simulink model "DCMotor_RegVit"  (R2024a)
settings: Solver=ode45  StartTime=0.0  StopTime=6  FixedStep=TE/100  RelTol=1e-3
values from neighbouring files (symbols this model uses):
  Ki = 0    [Constants_RegVit.m]
  Kp = 0    [Constants_RegVit.m]
  Kwc1 = 0    [Constants_RegVit.m]
  Kwc2 = 0    [Constants_RegVit.m]
  LIMREG = 0    [Constants_RegVit.m]
  TE = 0    [Constants_RegVit.m]
  TM = 0    [Constants_RegVit.m]
  TpE = 0    [Constants_RegVit.m]

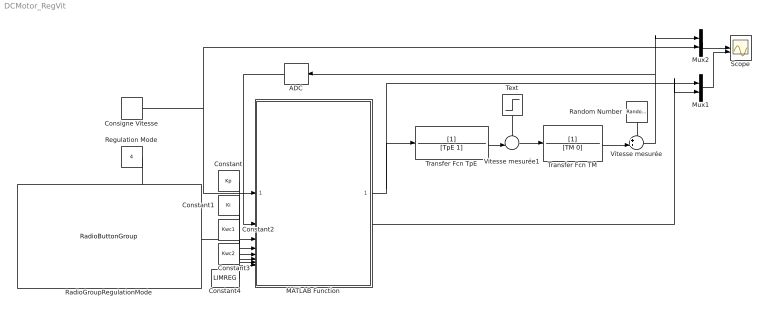
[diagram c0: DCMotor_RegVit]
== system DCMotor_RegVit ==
  ADC : ZeroOrderHold  SampleTime=TE
  Consigne Vitesse : DiscretePulseGenerator  Period=3/TE  PulseWidth=3/(2*TE)  SampleTime=TE
  Constant : Constant  Value=Kp
  Constant1 : Constant  Value=Ki
  Constant2 : Constant  Value=Kwc1
  Constant3 : Constant  Value=Kwc2
  Constant4 : Constant  Value=LIMREG
  MATLAB Function : MATLAB Function  TreatAsAtomicUnit=on
  Mux1 : Mux  Inputs=2
  Mux2 : Mux  Inputs=2
  RadioGroupRegulationMode : RadioButtonGroup  LabelPosition=Hide  SelectedLabel=THEORETICAL  ButtonGroupName=Regulation Mode
  Random Number : RandomNumber  Variance=0.00005  SampleTime=TE
  Regulation Mode : Constant  Value=4
  Scope : Scope  NumInputPorts=2
  Text : Step  Time=4  SampleTime=0
  Transfer Fcn TM : TransferFcn  Denominator=[TM 0]
  Transfer Fcn TpE : TransferFcn  Denominator=[TpE 1]
  Vitesse mesurée : Sum  Inputs=++|
  Vitesse mesurée1 : Sum  Inputs=-+|
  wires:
  Mux2/1 -> Scope/1
  Consigne Vitesse/1 -> Mux2/2, MATLAB Function/1(speedSetValue)
  Transfer Fcn TM/1 -> Vitesse mesurée/2
  Vitesse mesurée/1 -> Mux2/1, ADC/1
  Random Number/1 -> Vitesse mesurée/1
  ADC/1 -> MATLAB Function/2(speedMeasure)
  MATLAB Function/1(regOutLim) -> Mux1/1, Transfer Fcn TpE/1
  MATLAB Function/2(integratorOut) -> Mux1/2
  Mux1/1 -> Scope/2
  Transfer Fcn TpE/1 -> Vitesse mesurée1/2
  Vitesse mesurée1/1 -> Transfer Fcn TM/1
  Text/1 -> Vitesse mesurée1/1
  Constant3/1 -> MATLAB Function/7(Kwc2)
  Constant2/1 -> MATLAB Function/6(Kwc1)
  Constant1/1 -> MATLAB Function/5(Ki)
  Constant/1 -> MATLAB Function/4(Kp)
  Regulation Mode/1 -> MATLAB Function/3(regulationMode)
  Constant4/1 -> MATLAB Function/8(LIMREG)

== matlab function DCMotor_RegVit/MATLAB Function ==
function [regOutLim, integratorOut]  = fcn(speedSetValue, speedMeasure, regulationMode, Kp, Ki, Kwc1, Kwc2, LIMREG)
%% v02 : avec Théorique
%% constants definition
STANDARD    = 0;   % Standard mode (no ARW, no Cor)
GLOBAL      = 1;   % Global mode for the controller (ARW + Cor)
ARW         = 2;   % Anti-reset Windup mode (only ARW)
CORRECTOR   = 3;   % Corrector mode (only Cor)
THEORETICAL = 4;   % Theoretical mode (no ARW, no Cor, no Limitation)

% initialisation - DO NOT EDIT --------------------------------------------
persistent wc
if isempty(wc)
    wc = 0;
end
persistent integrator
if isempty(integrator)
    integrator = 0;
end


%% TO BE COMPLETED BY THE STUDENT -----------------------------------------

%% correcteur de consigne
% if (regulationMode == GLOBAL || regulationMode == CORRECTOR)
% else   
% end

%% Control
% your code here ...

%%ARW
% if (regulationMode == GLOBAL || regulationMode == ARW)
% 
% end


%% Integrator
% your code here ...



%% DO NOT EDIT ------------------------------------------------------------
integratorOut = integrator; % Integrator Output for display
